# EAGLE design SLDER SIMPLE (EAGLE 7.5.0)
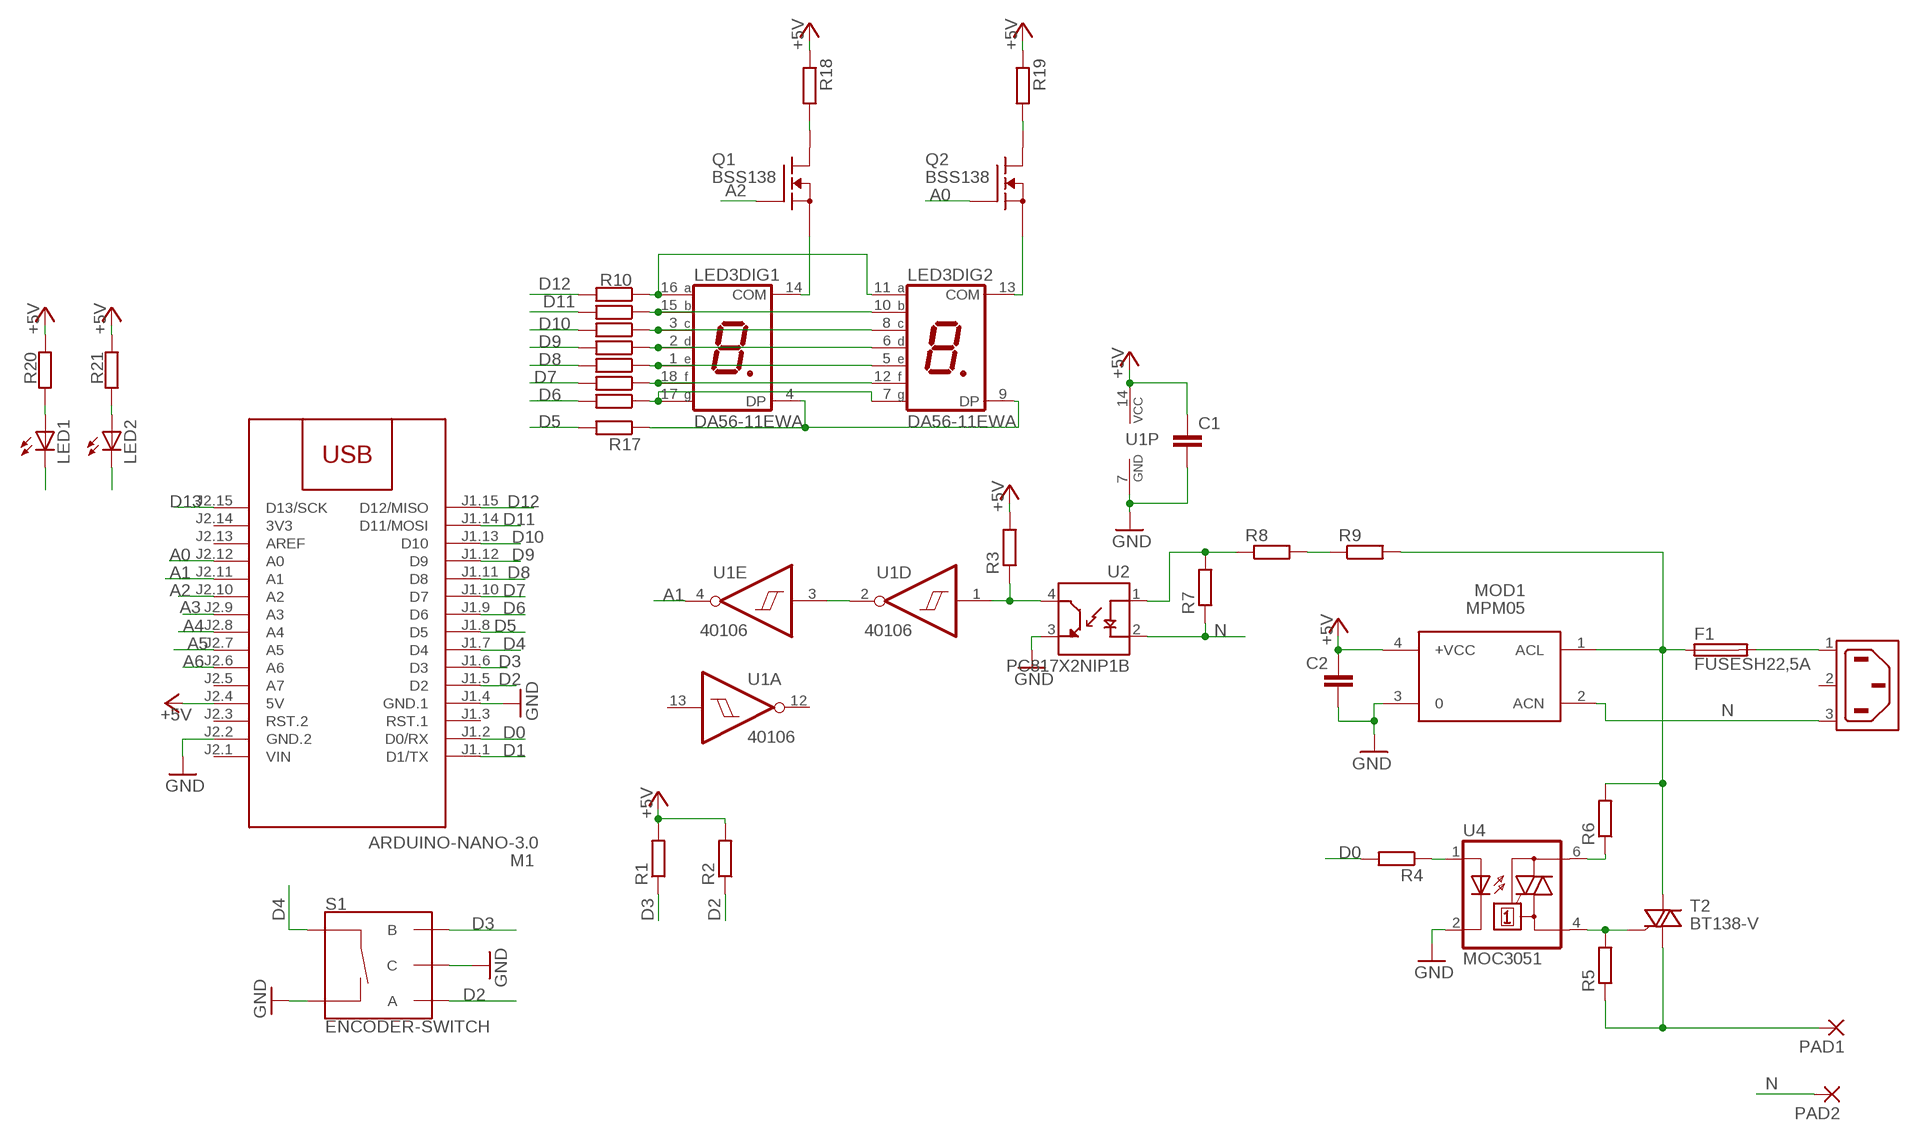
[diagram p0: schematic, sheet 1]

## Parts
C1  C-EUC1206  [C1206]
C2  C-EUC1206  [C1206]
F1  FUSESH22,5A  [SH22,5A]
LED1  LED5MM  [LED5MM]
LED2  LED5MM  [LED5MM]
LED3  DA56-11EWA  [DA56]
M1  ARDUINO-NANO-3.0  [ARDUINO-NANO-3.0]
MOD1  MPM05  [MPM05]
PAD1  3,17/1,3  [3,17/1,3]
PAD2  3,17/1,3  [3,17/1,3]
Q1  BSS138  [SOT23]
Q2  BSS138  [SOT23]
R1  R-EU_R1206  [R1206]
R2  R-EU_R1206  [R1206]
R3  R-EU_R1206  [R1206]
R4  R-EU_R1206  [R1206]
R5  R-EU_R1206  [R1206]
R6  R-EU_R1206  [R1206]
R7  R-EU_R2512  [R2512]
R8  R-EU_R2512  [R2512]
R9  R-EU_R2512  [R2512]
R10  R-EU_R1206  [R1206]
R11  R-EU_R1206  [R1206]
R12  R-EU_R1206  [R1206]
R13  R-EU_R1206  [R1206]
R14  R-EU_R1206  [R1206]
R15  R-EU_R1206  [R1206]
R16  R-EU_R1206  [R1206]
R17  R-EU_R1206  [R1206]
R18  R-EU_R1206  [R1206]
R19  R-EU_R1206  [R1206]
R20  R-EU_R1206  [R1206]
R21  R-EU_R1206  [R1206]
S1  ENCODER-SWITCH  [ROTARY_ENC_PLAIN]
T2  BT138-V  [TO220BV]
U1  40106  74HC14D  [SO14]
U2  PC817X2NIP1B  [SOIC254P960X420-4N]
U4  MOC3051  MOC3042M  [DIL06]
X1  6ESRM-P  [6ESRM-P]

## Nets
+5V: C1.1 C2.1 M1.J2.4(5V) MOD1.4(+VCC) R1.2 R2.2 R3.2 R18.1 R19.1 R20.1 R21.1 U1.14(P:VCC)
A0: M1.J2.12(A0) Q2.3(G)
A1: M1.J2.11(A1) U1.4(E:O)
A2: M1.J2.10(A2) Q1.3(G)
A3: M1.J2.9(A3)
A4: M1.J2.8(A4)
A5: M1.J2.7(A5)
A6: M1.J2.6(A6)
D0: M1.J1.2(D0/RX) R4.2
D1: LED2.K(C) M1.J1.1(D1/TX)
D2: M1.J1.5(D2) R2.1 S1.A
D3: M1.J1.6(D3) R1.1 S1.B
D4: M1.J1.7(D4) S1.SW+
D5: M1.J1.8(D5) R17.2
D6: M1.J1.9(D6) R16.2
D7: M1.J1.10(D7) R15.2
D8: M1.J1.11(D8) R14.2
D9: M1.J1.12(D9) R13.2
D10: M1.J1.13(D10) R12.2
D11: M1.J1.14(D11/MOSI) R11.2
D12: M1.J1.15(D12/MISO) R10.2
D13: LED1.K(C) M1.J2.15(D13/SCK)
GND: C1.2 C2.2 M1.J1.4(GND.1) M1.J2.2(GND.2) MOD1.3 S1.C S1.SW- U1.7(P:GND) U2.3(ET) U4.2(C)
N: MOD1.2(ACN) PAD2.1(P) R7.1 U2.2(C) X1.3(AC2)
N$1: LED3.11(DIG2:A) LED3.16(DIG1:A) R10.1
N$2: LED3.10(DIG2:B) LED3.15(DIG1:B) R11.1
N$3: LED3.3(DIG1:C) LED3.8(DIG2:C) R12.1
N$4: LED3.2(DIG1:D) LED3.6(DIG2:D) R13.1
N$5: LED3.1(DIG1:E) LED3.5(DIG2:E) R14.1
N$6: LED3.12(DIG2:F) LED3.18(DIG1:F) R15.1
N$7: LED3.7(DIG2:G) LED3.17(DIG1:G) R16.1
N$8: LED3.4(DIG1:DP) LED3.9(DIG2:DP) R17.1
N$9: LED3.14(DIG1:COM) Q1.1(S)
N$10: F1.2 X1.1(AC1)
N$11: F1.1 MOD1.1(ACL) R6.2 R9.2 T2.T2(A2)
N$12: R6.1 U4.6(A2)
N$13: R5.2 T2.G U4.4(A1)
N$14: PAD1.1(P) R5.1 T2.T1(A1)
N$15: R7.2 R8.1 U2.1(A)
N$16: R8.2 R9.1
N$17: R3.1 U1.1(D:I) U2.4(CT)
N$18: U1.2(D:O) U1.3(E:I)
N$19: R4.1 U4.1(A)
N$20: LED3.13(DIG2:COM) Q2.1(S)
N$21: Q1.2(D) R18.2
N$22: Q2.2(D) R19.2
N$23: LED1.A R20.2
N$24: LED2.A R21.2
Unconnected: M1.J1.3(RST.1) M1.J2.3(RST.2) M1.J2.5(A7) M1.J2.13(AREF) U1.5(F:I) U1.6(F:O) U1.8(C:O) U1.9(C:I) U1.10(B:O) U1.11(B:I) U1.12(A:O) U1.13(A:I) X1.2(SH)

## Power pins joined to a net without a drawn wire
3V3: M1.J2.14(3V3)
VIN: M1.J2.1(VIN)

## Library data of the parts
C1 C2 = rcl:C-EU: CAPACITOR, European symbol
F1 = fuse:FUSE: Fuse; OC_FARNELL: unknown; OC_NEWARK: unknown
LED1 LED2 = led:LED: LED
LED3 = display-kingbright:DA56-11: 14.22mm (0.56INCH) DUAL DIGIT NUMERIC DISPLAYS Source: www.kingbright.com .. DA56-11SRWA.pdf; OC_FARNELL: unknown; OC_NEWARK: unknown
M1 = diy-modules:ARDUINO-NANO-3.0: Arduino Nano 3.0 and compatible devices More details available here: https://www.arduino.cc/en/Main/ArduinoBoardNano Click here to find device on ebay.com
MOD1 = acdc:MPM05: AC DC Converter 5W
PAD1 PAD2 = wirepad:3,17/1,3: THROUGH-HOLE PAD
Q1 Q2 = transistor-fet:BSS138
R1-R21 = rcl:R-EU_: RESISTOR, European symbol
S1 = SparkFun-Switches:ENCODER-SWITCH: Rotary Encoder w/ Select Switch Encoders rotate similarly to potentiometers, but they’re different from potentiometers in that an encoder has full rotation without limits. They output gray code so that you can tell how much and in which direction the encoder has been turned. This encoder includes a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; SF_SKU: COM-09117
T2 = triac:BT138: TRIAC Source: http://www.semiconductors.philips.com BT138_SERIES_2.pdf
U1 = 74xx-eu:74*14: Hex schmitt trigger INVERTER
U2 = PC817X2NIP1B:PC817X2NIP1B: Check availability; AVAILABILITY: In Stock; CHECK_PRICES: https://www.snapeda.com/parts/PC817X2NIP1B/Sharp/view-part/?ref=eda; DESCRIPTION: Optocoupler DC-IN 1-CH Transistor DC-OUT 4-Pin DIP SMD T/R; MF: Sharp Microelectronics; MP: PC817X2NIP1B; PACKAGE: SMD-4 Sharp Microelectronics; PRICE: None; SNAPEDA_LINK: https://www.snapeda.com/parts/PC817X2NIP1B/Sharp/view-part/?ref=snap
U4 = optocoupler:MOC30*: 6-Pin DIP Zero-Cross Optoisolators Triac Driver Output (250/400 Volt Peak) Source: The old path of data sheet not more available 2013-05-06.; MF: FAIRCHILD SEMICONDUCTOR; MPN: MOC3042-M; OC_FARNELL: 1021368; OC_NEWARK: 72K8899
X1 = 6ESRM-P:6ESRM-P: Check availability; AVAILABILITY: In Stock; CHECK_PRICES: https://www.snapeda.com/parts/6ESRM-P/TE+Connectivity+Corcom+Filters/view-part/?ref=eda; COMMENT: 1609078-1; DESCRIPTION: AC Male Power Inlet Connector, PC Board Pins, Snap-In, 120/250VAC, 15A(UL/CSA), 10A; EU_ROHS_COMPLIANCE: Compliant; MF: TE Connectivity; MP: 6ESRM-P; PACKAGE: None; PRICE: None; SNAPEDA_LINK: https://www.snapeda.com/parts/6ESRM-P/TE+Connectivity+Corcom+Filters/view-part/?ref=snap

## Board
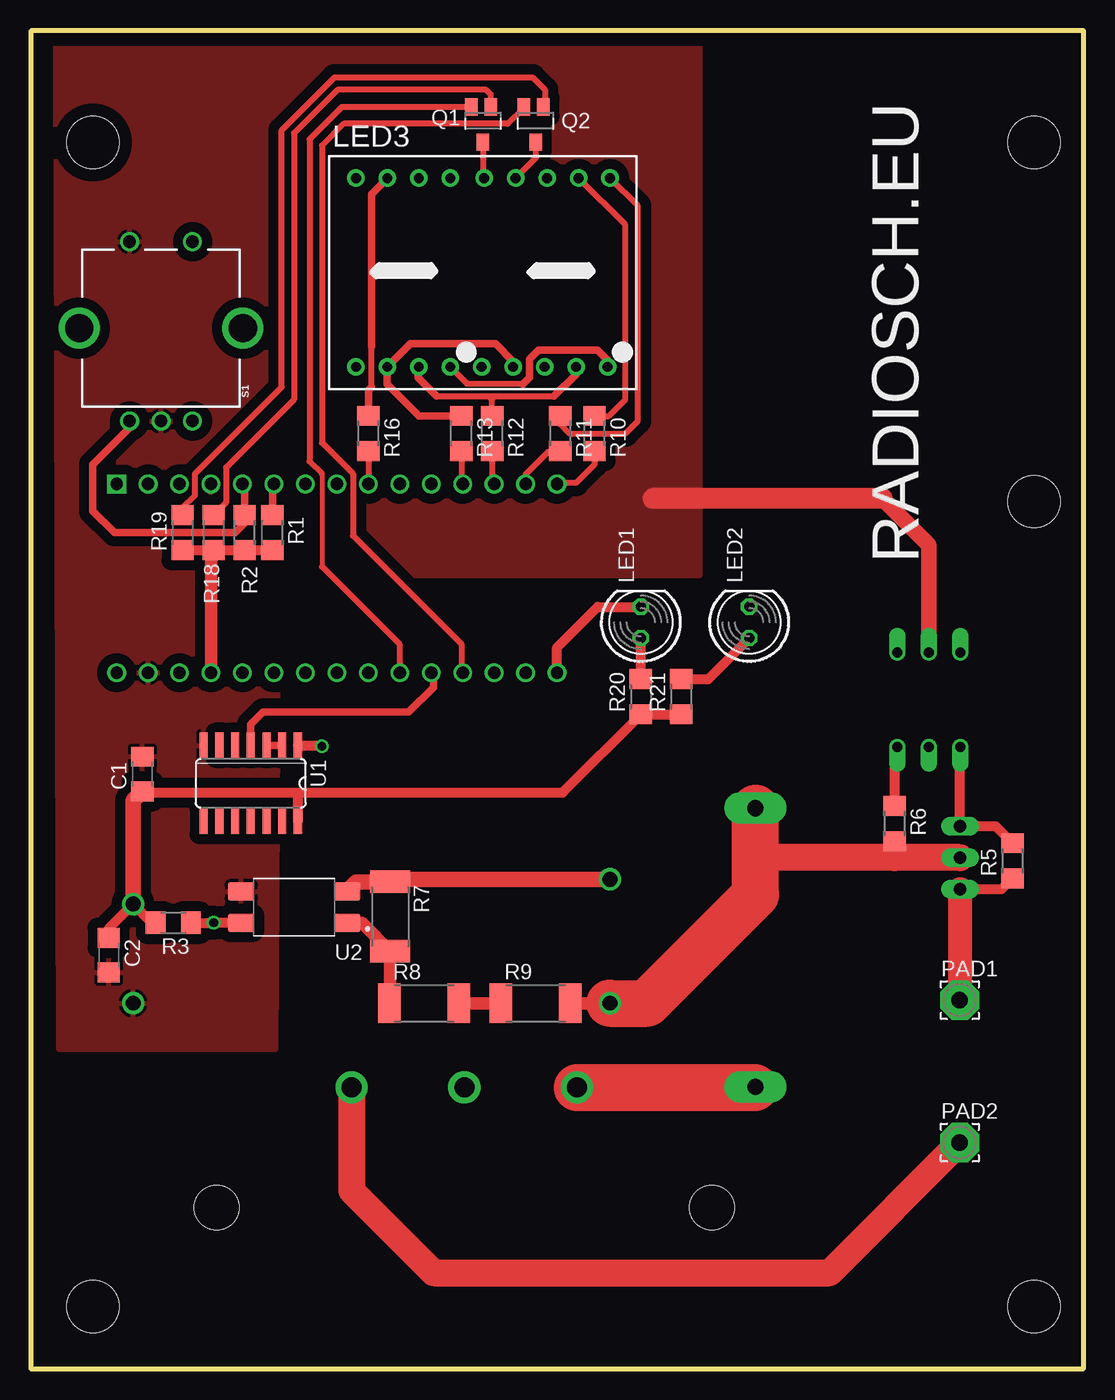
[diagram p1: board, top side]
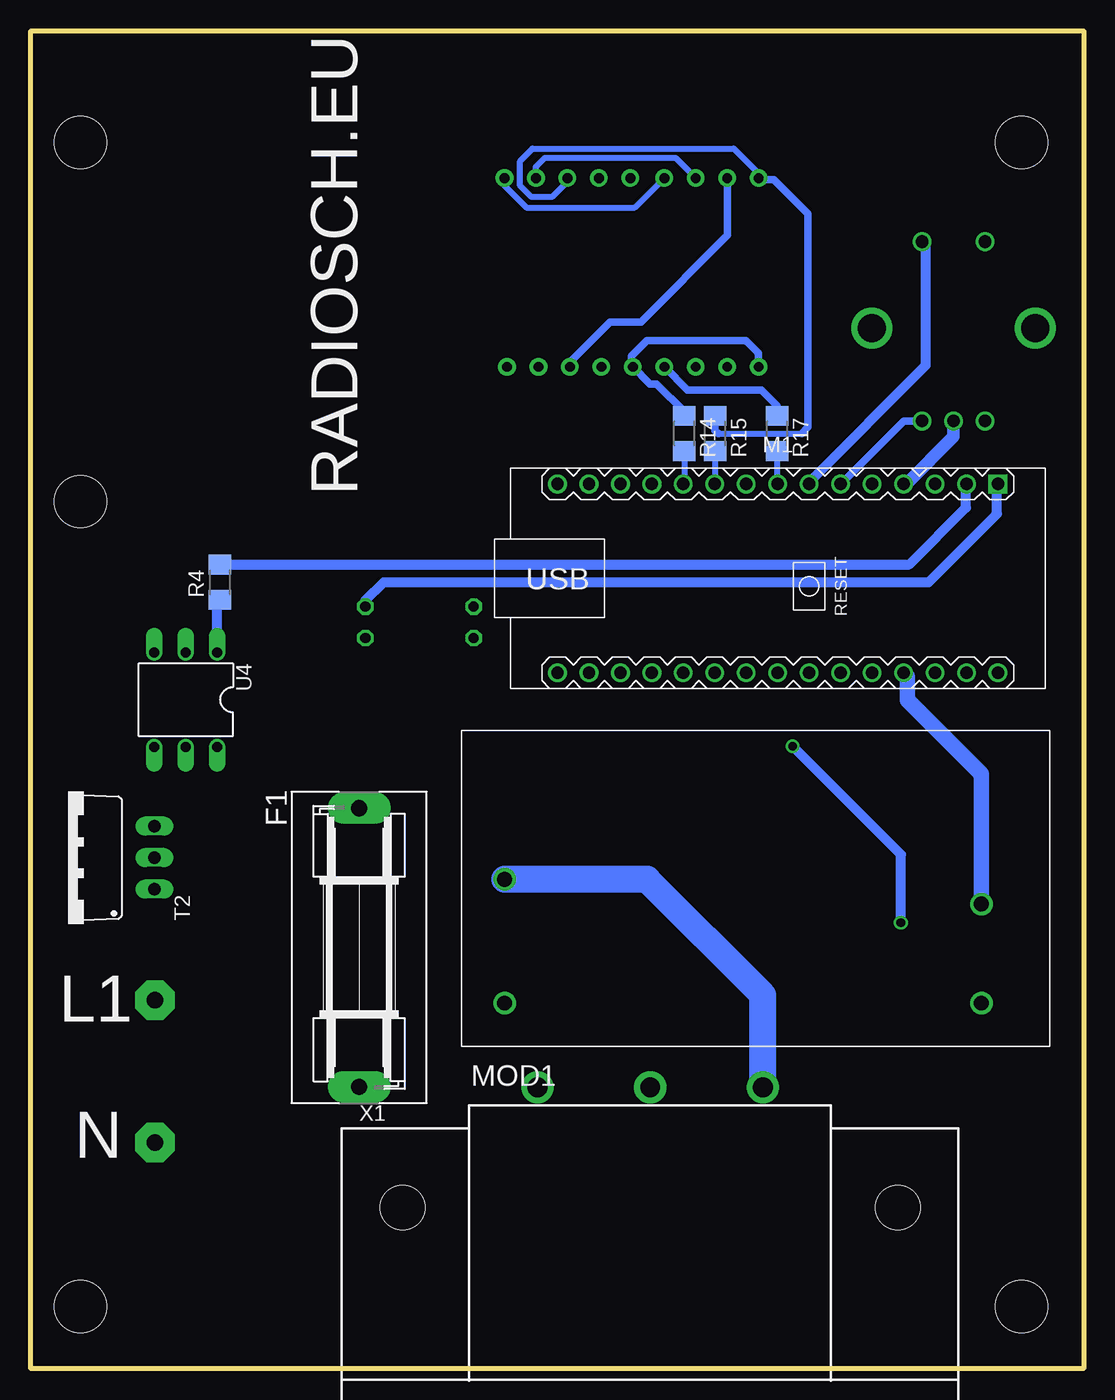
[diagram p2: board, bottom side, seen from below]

Size 85 x 108 mm. Coordinates in mm from the lower left corner, seen from the top.
Outline: 0,0 85,0 85,108 0,108 0,0
Copper layers (1*16): Top 0.035mm / dielectric 1.5mm / Bottom 0.035mm
Design rules "default": minimum track width 10mil, minimum drill 24mil, track to track 8mil, track to pad 8mil, pad to pad 8mil, via to via 8mil, smd to smd 8mil, copper to edge 40mil, drill to drill 8mil, minimum pad ring 10mil, minimum via ring 8mil, stop-mask expansion 4mil, vias tented up to drill 0mil, thermal gap 10mil
Holes 4.2 mm at 5,99 5,5 81,99 81,5 81,70

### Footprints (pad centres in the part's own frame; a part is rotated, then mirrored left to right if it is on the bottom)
C1206 = smd 1.6 x 1.8: 1 -1.4,0; 2 1.4,0
SH22,5A = drill 1.321 pad 2.54 long: 1 -11.252,0; 2 11.252,0
LED5MM = drill 0.813 octagon: A -1.27,0; K 1.27,0
DA56 = drill 0.8 pad 1.422: 1 -10.26,-7.62; 2 -7.72,-7.62; 3 -5.18,-7.62; 4 -2.64,-7.62; 5 -0.1,-7.62; 6 2.44,-7.62; 7 4.98,-7.62; 8 7.52,-7.62; 9 10.06,-7.62; 10 10.26,7.62; 11 7.72,7.62; 12 5.18,7.62; 13 2.64,7.62; 14 0.1,7.62; 15 -2.64,7.62; 16 -5.18,7.62; 17 -7.72,7.62; 18 -10.26,7.62
ARDUINO-NANO-3.0 = drill 1 square: J1.1 17.78,7.62 | drill 1: J1.2 15.24,7.62; J1.3 12.7,7.62; J1.4 10.16,7.62; J1.5 7.62,7.62; J1.6 5.08,7.62; J1.7 2.54,7.62; J1.8 0,7.62; J1.9 -2.54,7.62; J1.10 -5.08,7.62; J1.11 -7.62,7.62; J1.12 -10.16,7.62; J1.13 -12.7,7.62; J1.14 -15.24,7.62; J1.15 -17.78,7.62; J2.1 17.78,-7.62; J2.2 15.24,-7.62; J2.3 12.7,-7.62; J2.4 10.16,-7.62; J2.5 7.62,-7.62; J2.6 5.08,-7.62; J2.7 2.54,-7.62; J2.8 0,-7.62; J2.9 -2.54,-7.62; J2.10 -5.08,-7.62; J2.11 -7.62,-7.62; J2.12 -10.16,-7.62; J2.13 -12.7,-7.62; J2.14 -15.24,-7.62; J2.15 -17.78,-7.62
MPM05 = drill 1.2: 1 3.5,-22; 2 3.5,-12; 3 42,-22; 4 42,-14
3,17/1,3 = drill 1.321 pad 3.175 octagon: 1 0,0
SOT23 = smd 1 x 1.4: 1 0,1.735; 2 -0.632,-1.1; 3 0.95,-1.1
R1206 = smd 1.6 x 1.803: 1 -1.422,0; 2 1.422,0
R2512 = smd 1.8 x 3.2: 1 -2.8,0; 2 2.8,0
ROTARY_ENC_PLAIN = drill 1.016: A 7.493,-2.54; B 7.493,2.54; C 7.493,0; SW+ -6.985,2.54; SW- -6.985,-2.54 | drill 2.286: P$3 0,6.604; P$4 0,-6.604
TO220BV = drill 1.016 long: G 2.54,-6.985; T1 -2.54,-6.985; T2 0,-6.985
SO14 = smd 0.66 x 2.032: 1 -3.81,-3.073; 2 -2.54,-3.073; 3 -1.27,-3.073; 4 0,-3.073; 5 1.27,-3.073; 6 2.54,-3.073; 7 3.81,-3.073; 8 3.81,3.073; 9 2.54,3.073; 10 1.27,3.073; 11 0,3.073; 12 -1.27,3.073; 13 -2.54,3.073; 14 -3.81,3.073
SOIC254P960X420-4N = smd 2.15 x 1.48: 1 -4.28,1.27; 2 -4.28,-1.27; 3 4.28,-1.27; 4 4.28,1.27
DIL06 = drill 0.813 offset: 1 -2.54,-3.81; 2 0,-3.81; 3 2.54,-3.81; 4 2.54,3.81; 5 0,3.81; 6 -2.54,3.81
6ESRM-P = drill 1.6 pad 2.6: 1 -9.1,9.7; 2 0,9.7; 3 9.1,9.7 | hole 3.6: -20,0; 20,0

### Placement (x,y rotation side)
C1  9,48 90 top
C2  6.28,33.38 270 top
F1  58.5,34 270 bottom
LED1  49.25,60.25 90 top
LED2  58,60.25 90 top
LED3  36.5,88.5 0 top
M1  24.7,63.8 0 bottom
MOD1  50.25,51.5 0 bottom
PAD1  75,29.75 0 top
PAD2  75,18.25 0 top
Q1  36.5,100.75 180 top
Q2  40.75,100.75 180 top
R1  19.5,67.5 270 top
R2  17.25,67.5 270 top
R3  11.5,36 180 top
R4  69.75,63.5 90 bottom
R5  79.25,41 90 top
R6  69.75,44 270 top
R7  29,36.5 270 top
R8  31.75,29.5 0 top
R9  40.75,29.5 0 top
R10  45.5,75.5 270 top
R11  42.75,75.5 270 top
R12  37.25,75.5 270 top
R13  34.75,75.5 270 top
R14  32.25,75.5 270 bottom
R15  29.75,75.5 270 bottom
R16  27.25,75.5 270 top
R17  24.75,75.5 270 bottom
R18  14.75,67.5 90 top
R19  12.25,67.5 90 top
R20  49.25,54.25 90 top
R21  52.5,54.25 90 top
S1  10.5,84 270 top
T2  82,41.25 90 bottom
U1  17.75,47.25 180 top
U2  21.25,37.25 180 top
U4  72.5,54 180 bottom
X1  35,13 0 bottom

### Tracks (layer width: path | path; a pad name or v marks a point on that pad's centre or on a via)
+5V
  Top 0.813: R19.1 R18.1 15.25,66.08 R2.2 R1.2 | U1.14 21.56,46.19 21.25,46.5 | C1.1 9.1,46.5 21.25,46.5 | C2.1 6.28,35.53 MOD1.4 9.75,36 R3.2 | 21.25,46.5 42.92,46.5 R20.1 R21.1
  Top 1.016: M1.J2.4 14.54,65.37 15.25,66.08
  Top 1.27: MOD1.4 8.25,45.85 C1.1
  Bottom 1.27: MOD1.4 8.25,48 14.25,54 14.25,55.89 M1.J2.4
A0
  Top 0.5: Q2.3 39.8,101.8 38.5,100.5 25.25,100.5 23.5,98.75 23.5,74.75 26,72.25 26,67.25 34.75,58.5 34.75,56.29 M1.J2.12
A1
  Top 0.61: U1.4 17.75,52 18.75,53 30.5,53 32.5,55 32.5,56 M1.J2.11
A2
  Top 0.406: 23.5,72.25 23.5,64.75
  Top 0.5: Q1.3 25.1,101.85 22.5,99.25 22.5,73.25 23.5,72.25 | 23.5,64.75 29.75,58.5 29.75,56.21 M1.J2.10
D0
  Bottom 0.813: R4.2 14.08,64.92 9.5,69.5 9.5,71.38 M1.J1.2
D1
  Bottom 0.813: LED2.K 58,62 56.5,63.5 12.5,63.5 7,69 7,71.34 M1.J1.1
D2
  Top 0.61: M1.J1.5 17.25,71.25 R2.1 17.25,68.25 16.5,67.5 6.75,67.5 5,69.25 5,73 7.96,75.96 S1.A
D3
  Top 0.61: R1.1 19.5,71.3 M1.J1.6
  Bottom 0.61: M1.J1.6 19.58,71.42 14.5,76.5 S1.B
D4
  Bottom 0.813: M1.J1.7 22.16,71.59 12.75,81 12.75,90.69 S1.SW+
D5
  Bottom 0.5: R17.2 24.75,71.47 M1.J1.8
D6
  Top 0.5: R16.2 M1.J1.9
D7
  Bottom 0.5: R15.2 29.75,71.45 M1.J1.10
D8
  Bottom 0.5: R14.2 32.25,71.49 M1.J1.11
D9
  Top 0.5: R13.2 34.75,71.53 M1.J1.12
D10
  Top 0.5: R12.2 37.25,71.57 M1.J1.13
D11
  Top 0.5: M1.J1.14 39.94,72.19 41.75,74 42.67,74 R11.2
D12
  Top 0.5: R10.2 45.5,73 44,71.5 42.56,71.5 M1.J1.15
D13
  Top 0.813: M1.J2.15 42.48,58.23 45.75,61.5 49.23,61.5 LED1.K
GND
  Top 1.016: 50.25,70.25 50,70
  Top 1.27: U4.2 72.5,66.5 68.75,70.25
  Top 1.676: 68.75,70.25 50.25,70.25
  Bottom 1.016: M1.J1.4 14.33,71.42 10.5,75.25 S1.C
  pour Top (isolate 0.813): 19.75,25.75 2.25,25.75 2,107 54,107 54,64 20,64
N
  Top 1.27: MOD1.2 29.2,39.5 R7.1 26.31,39.3 U2.2
  Top 2.184: X1.3 25.9,14.35 32.5,7.75 64.5,7.75 PAD2.1
  Bottom 2.184: X1.3 25.9,30.15 35.25,39.5 MOD1.2
N$1
  Top 0.5: R10.1 46.67,76.92 48,78.25 48,92.34 LED3.11
  Bottom 0.5: LED3.11 44.22,97.03 43.5,97.75 32.95,97.75 LED3.16
N$2
  Top 0.5: R11.1 42.75,76.25 43.5,75.5 48,75.5 49,76.5 49,93.88 LED3.10
  Bottom 0.5: LED3.10 46.76,95.51 45,93.75 36.23,93.75 LED3.15
N$3
  Top 0.5: 32.75,78.5 37,78.5 | 37,78.5 42.25,78.5 | R12.1 37.25,78.25 37,78.5
  Top 0.61: 32.75,78.5 31.25,80 31.25,80.81 LED3.3 | LED3.8 44.02,80.27 42.25,78.5
N$4
  Top 0.61: R13.1 31.33,76.92 28.75,79.5 28.75,80.85 LED3.2 30.65,82.75 37.5,82.75 38.94,81.31 LED3.6
N$5
  Bottom 0.61: R14.1 32.25,77.25 34.5,79.5 35.02,79.5 LED3.5 36.5,80.98 36.5,81.75 35.25,83 27.25,83 26.24,81.99 LED3.1
N$6
  Bottom 0.5: 29.5,75.5 22.75,75.5 | LED3.12 41.68,95.82 42.88,94.62 44.62,94.62 45.5,95.5 45.5,97.5 44.5,98.5 28.25,98.5 25.75,96
  Bottom 0.61: R15.1 29.75,75.75 29.5,75.5 | 22.75,75.5 22.25,76 22.25,93.25 25,96 25.75,96 26.12,96 LED3.18
N$7
  Top 0.5: 27.5,79.25 27.5,82.5
  Top 0.61: R16.1 27.25,79 27.5,79.25 | 27.5,82.5 27.5,94.84 LED3.17
  Bottom 0.61: LED3.7 41.48,81.27 38.25,84.5 35.75,84.5 28.75,91.5 28.75,96.09 LED3.17
N$8
  Top 0.5: 39.75,79.5 35.24,79.5 LED3.4
  Top 0.61: LED3.9 46.56,81.44 45.75,82.25 41,82.25 40.25,81.5 40.25,80 39.75,79.5
  Bottom 0.61: R17.1 24.75,77.75 26,79 31.98,79 LED3.4
N$9
  Top 0.5: Q1.1 36.5,96.22 LED3.14
N$10
  Top 2.184: 58.45,22.7 F1.2
  Top 3.81: X1.1 58.45,22.7
N$11
  Top 1.016: MOD1.1 R9.2 | R6.2 69.75,41.25
  Top 2.184: T2.T2 69.75,41.25 58.75,41.25 58.5,41.5
  Top 3.81: MOD1.1 49.75,29.5 58.5,38.25 58.5,41.5 F1.1
N$12
  Top 0.813: R6.1 69.75,49.98 U4.6
N$13
  Top 0.813: U4.4 75.02,50.16 T2.G 77.88,43.79 R5.2
N$14
  Top 0.813: T2.T1 78.38,38.71 R5.1
  Top 1.93: T2.T1 75.02,29.77 PAD1.1
N$15
  Top 1.016: U2.1 26.72,35.98 R7.2 29,29.55 R8.1
N$16
  Top 1.016: R8.2 R9.1
N$17  (via drill 0.7)
  Top 0.813: R3.1 v14.75,36 14.77,35.98 U2.4 | v23.5,50.25 21.63,50.25 U1.1
  Bottom 0.813: v23.5,50.25 14.75,41.5 v14.75,36
N$18
  Top 0.61: U1.3 U1.2
N$19
  Bottom 0.813: U4.1 69.96,61.87 R4.1
N$20
  Top 0.5: Q2.1 40.75,97.73 LED3.13
N$21
  Top 0.5: Q1.2 37.13,102.87 36.75,103.25 24.75,103.25 21.25,99.75 21.25,78.25 15.75,72.75 15.75,69.92 R18.2
N$22
  Top 0.5: R19.2 12.25,69.5 13.25,70.5 13.25,72.25 20.25,79.25 20.25,100 24.5,104.25 40.5,104.25 41.5,103.25 41.5,101.97 Q2.2
N$23
  Top 0.813: R20.2 LED1.A
N$24
  Top 0.813: R21.2 54.69,55.67 LED2.A

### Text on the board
tPlace: RADIOSCH.EU
bPlace: RADIOSCH.EU | L1 | N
